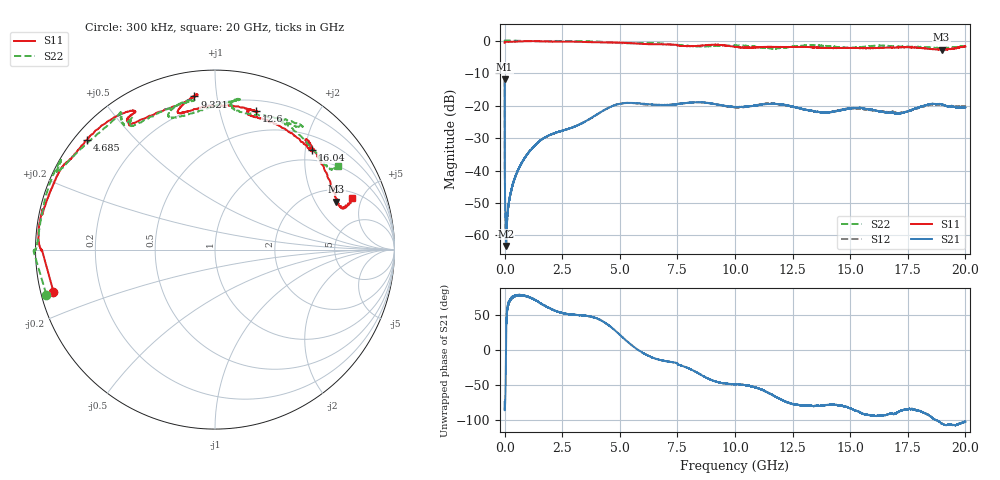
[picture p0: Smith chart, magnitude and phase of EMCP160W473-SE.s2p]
!EMCP160W473
!Johanson Technology Inc.
!www.johansontechnology.com
!Test Board Conditions:
!Substrate Type  RO4350B
!Substrate Thickness  10 mil
!Substrate Dk  3.66
!TL Type: GCPW
!TL Trace Width  20 mil
!TL Gap  10 mil
!PART MODE SINGLE ENDED (AKA BYPASS)
!DUT TOPOLOGY	SERIES-SHUNT
# MHz S  dB  R 50
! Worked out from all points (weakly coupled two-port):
!   20001 points, 300 kHz to 20 GHz, reference 50 ohm
!   highest |S21| = -11.85 dB at 300 kHz (marker M1); lowest = -63.3 dB at 59.3 MHz (marker M2)
!   lowest |S11| = -2.8 dB at 18.97 GHz (marker M3), VSWR 6.33, Z = 134 + j152 ohm
!   |S11| at or under -10 dB: nowhere
!   |S22| runs from -2.4 to 0.1 dB; largest |S21 - S12| = 0.0056
!   S11 on the Smith chart (normalised r, x): 300 kHz: 0.04, -0.13; 4.685 GHz: 0.03, +0.37; 9.321 GHz: 0.13, +0.87; 12.6 GHz: 0.30, +1.30; 16.04 GHz: 0.77, +2.13; 20 GHz: 2.42, +4.18
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0.3  -0.63 -165.4  -11.85 -74.7  -11.89 -74.9  -0.24 -165.1
59.299  -0.32 -179.9  -63.25 -13.3  -62.62 -10.3  0.08 -179.9
122.298  -0.32 -179.8  -53.86 58.0  -53.80 58.6  0.06 -179.9
430.294  -0.27 179.9  -42.58 75.7  -42.57 76.9  0.03 -179.8
1081.284  -0.11 174.1  -34.10 74.7  -34.04 74.5  -0.10 176.8
2318.265  -0.26 157.3  -28.14 53.8  -28.15 54.1  -0.05 152.3
3334.25  -0.33 150.1  -25.51 48.9  -25.50 48.8  -0.11 152.1
4685.23  -0.53 139.4  -20.12 30.4  -20.08 30.8  -0.55 144.3
6667.2  -1.07 121.6  -19.76 -13.9  -19.82 -13.4  -0.74 124.8
7455.188  -1.25 124.2  -19.63 -18.9  -19.60 -18.9  -1.27 126.1
8184.177  -1.65 107.7  -19.00 -29.7  -19.02 -29.7  -1.66 123.1
9321.16  -1.30 97.7  -19.75 -46.9  -19.77 -47.4  -1.58 101.1
10000.15  -1.85 104.4  -20.39 -49.2  -20.54 -49.4  -1.48 98.6
11257.13  -1.91 88.3  -19.58 -58.3  -19.46 -58.5  -2.14 108.8
12599.11  -1.90 73.5  -20.47 -78.0  -20.55 -77.9  -1.73 85.9
13334.1  -1.99 76.6  -21.58 -80.1  -21.62 -79.8  -1.44 80.8
14700.08  -2.21 66.5  -21.24 -80.7  -21.13 -80.7  -2.08 81.5
16042.06  -2.22 45.9  -21.40 -94.2  -21.47 -92.9  -1.53 57.2
16667.05  -2.13 47.9  -22.22 -91.9  -21.96 -90.9  -1.59 55.2
17760.03  -2.07 47.5  -21.03 -85.4  -21.11 -86.5  -1.89 62.6
18967.01  -2.77 21.5  -19.60 -105.2  -19.75 -103.4  -2.28 40.2
20000  -1.75 20.5  -20.50 -102.6  -20.11 -103.9  -1.64 34.3
